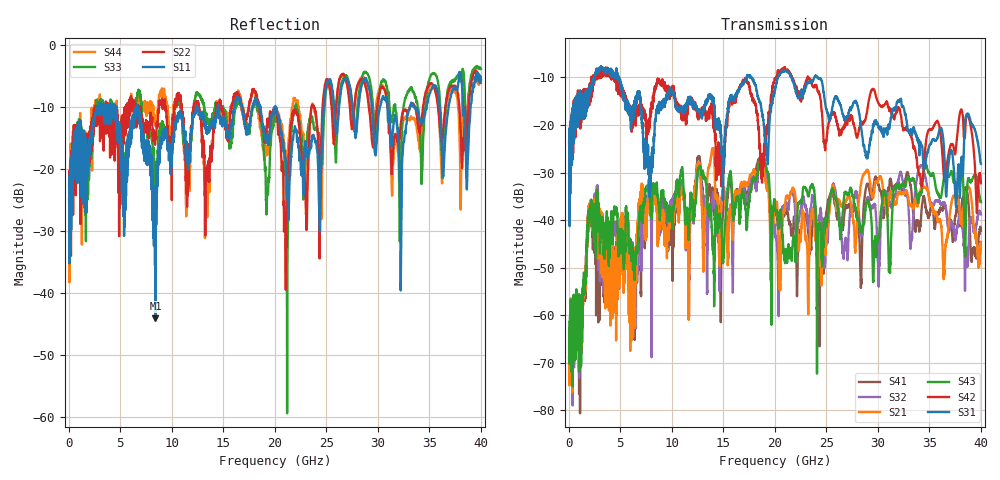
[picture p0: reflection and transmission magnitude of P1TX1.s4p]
!Agilent Technologies,N5245A,MY49151084,A.09.20.08
!Agilent N5245A: A.09.20.08
!Date: Thursday, March 01, 2012 13:10:06
!Correction: S11(Full 4 Port(1,2,3,4))
!S12(Full 4 Port(1,2,3,4))
!S13(Full 4 Port(1,2,3,4))
!S14(Full 4 Port(1,2,3,4))
!S21(Full 4 Port(1,2,3,4))
!S22(Full 4 Port(1,2,3,4))
!S23(Full 4 Port(1,2,3,4))
!S24(Full 4 Port(1,2,3,4))
!S31(Full 4 Port(1,2,3,4))
!S32(Full 4 Port(1,2,3,4))
!S33(Full 4 Port(1,2,3,4))
!S34(Full 4 Port(1,2,3,4))
!S41(Full 4 Port(1,2,3,4))
!S42(Full 4 Port(1,2,3,4))
!S43(Full 4 Port(1,2,3,4))
!S44(Full 4 Port(1,2,3,4))
!S4P File: Measurements: <S11,S12,S13,S14>,
!<S21,S22,S23,S24>,
!<S31,S32,S33,S34>,
!<S41,S42,S43,S44>:
# Hz S  dB  R 50
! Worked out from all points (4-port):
!   3996 points, 50 MHz to 40 GHz, reference 50 ohm
!   strongest paths, dB at 50 MHz, 10.04 GHz, 20.03 GHz, 30.02 GHz, 40 GHz:
!     S31: -23.6, -13.2, -12.6, -20.0, -28.1
!     S42: -24.2, -12.7, -10.3, -15.2, -32.2
!     S43: -66.9, -39.8, -37.3, -44.3, -36.2
!     S21: -69.9, -39.1, -36.7, -31.6, -44.5
!     S32: -68.8, -36.6, -42.3, -50.1, -38.8
!     S41: -68.7, -43.0, -38.3, -32.3, -42.2
!   lowest |S11| = -44.1 dB at 8.43 GHz (marker M1), VSWR 1.01, Z = 50.6 - j0.0127 ohm
!   |S11| at or under -10 dB: start of sweep to 2.868 GHz; 6.685 GHz to 12.38 GHz (5.692 GHz wide, 59.7 % of centre); 20.07 GHz to 24.77 GHz (4.699 GHz wide, 21 % of centre)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
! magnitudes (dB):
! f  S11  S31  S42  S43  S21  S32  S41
! 50 MHz  -23.2  -23.6  -24.2  -66.9  -69.9  -68.8  -68.7
! 2.07 GHz  -15.0  -12.5  -14.5  -38.2  -37.0  -37.2  -37.9
! 8.43 GHz  -44.1  -19.0  -11.9  -34.3  -35.4  -36.6  -33.6
! 18.77 GHz  -11.7  -17.3  -32.1  -27.0  -28.3  -27.3  -27.8
! 21.03 GHz  -18.2  -8.5  -8.2  -47.8  -36.2  -37.1  -37.9
! 25.05 GHz  -6.4  -17.2  -22.4  -40.7  -42.7  -43.5  -37.9
! 40 GHz  -6.1  -28.1  -32.2  -36.2  -44.5  -38.8  -42.2
